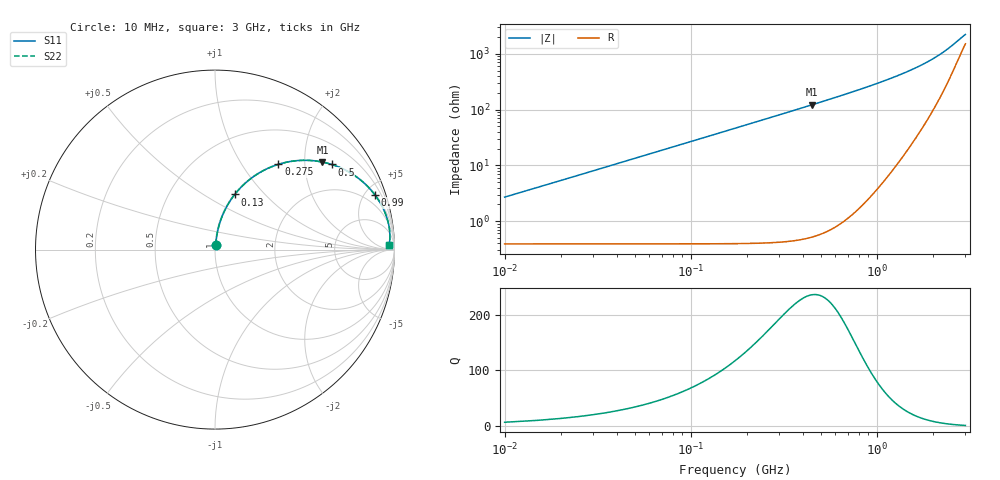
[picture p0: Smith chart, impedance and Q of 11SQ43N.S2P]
! Coilcraft 1111SQ-43N Air Core Inductor
! 15 MAR 2012
# MHZ S MA R 50
!Freq  MagS11  AngS11  MagS21  AngS21  MagS12  AngS12  MagS22  AngS22
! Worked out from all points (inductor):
!   599 points, 10 MHz to 3 GHz, reference 50 ohm
!   read as one part in series: L = 42.4 nH near 20 MHz
!   highest Q = 236 at 450 MHz (marker M1), where L = 43.2 nH
!   S11 on the Smith chart (normalised r, x): 10 MHz: 1.01, +0.05; 130 MHz: 1.01, +0.69; 275 MHz: 1.01, +1.47; 500 MHz: 1.01, +2.73; 990 MHz: 1.08, +5.81; 3 GHz: 38, +32
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10  0.02679 80.1  0.9958 -1.5  0.9958 -1.5  0.02679 80.1
15  0.03993 82.1  0.9953 -2.3  0.9953 -2.3  0.03993 82.1
25  0.06626 82.9  0.9939 -3.8  0.9939 -3.8  0.06626 82.9
30  0.0794 82.7  0.993 -4.6  0.993 -4.6  0.0794 82.7
40  0.1056 81.8  0.9906 -6.1  0.9906 -6.1  0.1056 81.8
55  0.1444 80.2  0.9857 -8.3  0.9857 -8.3  0.1444 80.2
85  0.22 76.3  0.9717 -12.7  0.9717 -12.7  0.22 76.3
130  0.3264 70.3  0.9416 -19.1  0.9416 -19.1  0.3264 70.3
195  0.4605 62.1  0.8841 -27.4  0.8841 -27.4  0.4605 62.1
275  0.5918 53.4  0.8028 -36.3  0.8028 -36.3  0.5918 53.4
355  0.6894 46.1  0.7212 -43.6  0.7212 -43.6  0.6894 46.1
450  0.7718 39.2  0.6325 -50.6  0.6325 -50.6  0.7719 39.2
500  0.8044 36.2  0.5907 -53.6  0.5907 -53.6  0.8044 36.2
510  0.8102 35.6  0.5827 -54.2  0.5827 -54.2  0.8102 35.6
610  0.8575 30.6  0.5104 -59.1  0.5104 -59.1  0.8575 30.6
720  0.8932 26.3  0.4443 -63.4  0.4443 -63.4  0.8932 26.3
990  0.9415 18.9  0.3259 -70.4  0.3259 -70.4  0.9415 18.9
1010  0.9437 18.5  0.319 -70.8  0.319 -70.8  0.9437 18.5
1505  0.9727 11.0  0.1944 -76.5  0.1944 -76.5  0.9727 11.0
2005  0.9786 6.6  0.1204 -76.6  0.1204 -76.6  0.9786 6.6
2505  0.9761 3.7  0.07218 -69.0  0.07218 -69.0  0.9761 3.7
3000  0.9698 1.5  0.04362 -45.6  0.04362 -45.6  0.9698 1.5
